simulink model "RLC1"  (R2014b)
settings: Solver=ode45  StartTime=0.0  StopTime=0.01  RelTol=1e-3
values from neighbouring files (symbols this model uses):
  C = [0 1 0 0;0 0 0 1]    [impuls_antw_zustand_1.m]    (also in impuls_antwort_1.m = 1e-07; impuls_antwort_2.m = 1e-07; impuls_antwort_3.m = 1e-07; impuls_antwort_4.m = 1e-07)
  fsig = 250    [einseitig_1.m]    (also in abtast_rate_1.m = 100; ad_test_12.m = ',num2str(fsig),'; ad_test_2.m = ',num2str(fsig),'; ad_test_3.m = ',num2str(fsig),')
  L = 0.01    [impuls_antwort_1.m]    (also in impuls_antwort_2.m; impuls_antwort_3.m; impuls_antwort_4.m; RLC_reihen_1.m)
  R = 50    [impuls_antwort_1.m]    (also in impuls_antwort_2.m; impuls_antwort_3.m; impuls_antwort_4.m; RLC_reihen_1.m)
  uc0 = -2    [RLC_reihen_1.m]    (also in RLC_reihen_3.m; RLC_reihen_4.m)
undefined symbols (not defined in the file or in its folder): vuc0

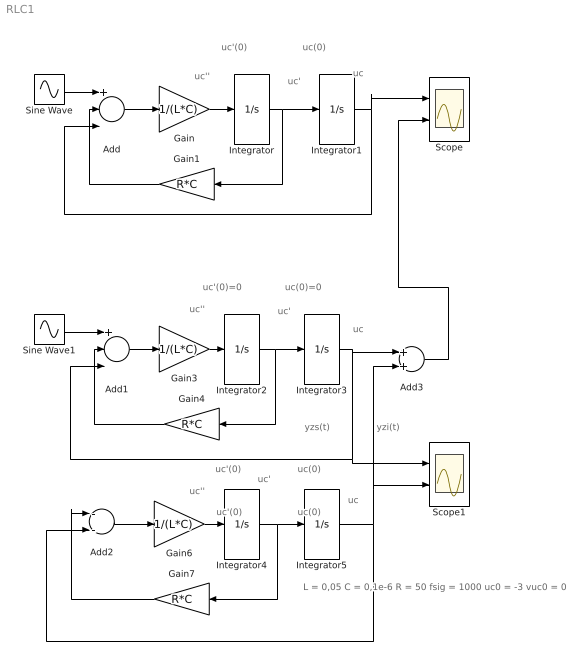
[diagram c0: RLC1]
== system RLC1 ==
  note: uc(0)
  note: uc'(0)
  note: yzs(t)
  note: yzi(t)
  note: L = 0,05 C = 0,1e-6 R = 50 fsig = 1000 uc0 = -3 vuc0 = 0
  note: uc(0)
  note: uc'(0)
  note: uc
  note: uc'
  note: uc''
  note: uc(0)=0
  note: uc'(0)=0
  note: uc
  note: uc'
  note: uc''
  note: uc(0)
  note: uc'(0)
  note: uc
  note: uc'
  note: uc''
  Add : Sum  Inputs=+--
  Add1 : Sum  Inputs=+--
  Add2 : Sum  Inputs=--
  Add3 : Sum
  Gain : Gain  Gain=1/(L*C)
  Gain1 : Gain  Gain=R*C
  Gain3 : Gain  Gain=1/(L*C)
  Gain4 : Gain  Gain=R*C
  Gain6 : Gain  Gain=1/(L*C)
  Gain7 : Gain  Gain=R*C
  Integrator : Integrator  InitialCondition=vuc0
  Integrator1 : Integrator  InitialCondition=uc0
  Integrator2 : Integrator
  Integrator3 : Integrator
  Integrator4 : Integrator  InitialCondition=vuc0
  Integrator5 : Integrator  InitialCondition=uc0
  Scope : Scope  NumInputPorts=2
  Scope1 : Scope  NumInputPorts=2
  Sine Wave : Sin  Frequency=2*pi*fsig  SampleTime=0
  Sine Wave1 : Sin  Frequency=2*pi*fsig  SampleTime=0
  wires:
  Sine Wave/1 -> Add/1
  Add/1 -> Gain/1
  Gain/1 -> Integrator/1
  Gain1/1 -> Add/2
  Integrator1/1 -> Scope/1, Add/3
  Sine Wave1/1 -> Add1/1
  Add1/1 -> Gain3/1
  Gain3/1 -> Integrator2/1
  Integrator2/1 -> Integrator3/1, Gain4/1
  Gain4/1 -> Add1/2
  Integrator3/1 -> Add3/1, Add1/3, Scope1/1
  Add2/1 -> Gain6/1
  Gain6/1 -> Integrator4/1
  Gain7/1 -> Add2/1
  Integrator5/1 -> Add2/2, Scope1/2, Add3/2
  Integrator/1 -> Gain1/1, Integrator1/1
  Add3/1 -> Scope/2
  Integrator4/1 -> Integrator5/1, Gain7/1
